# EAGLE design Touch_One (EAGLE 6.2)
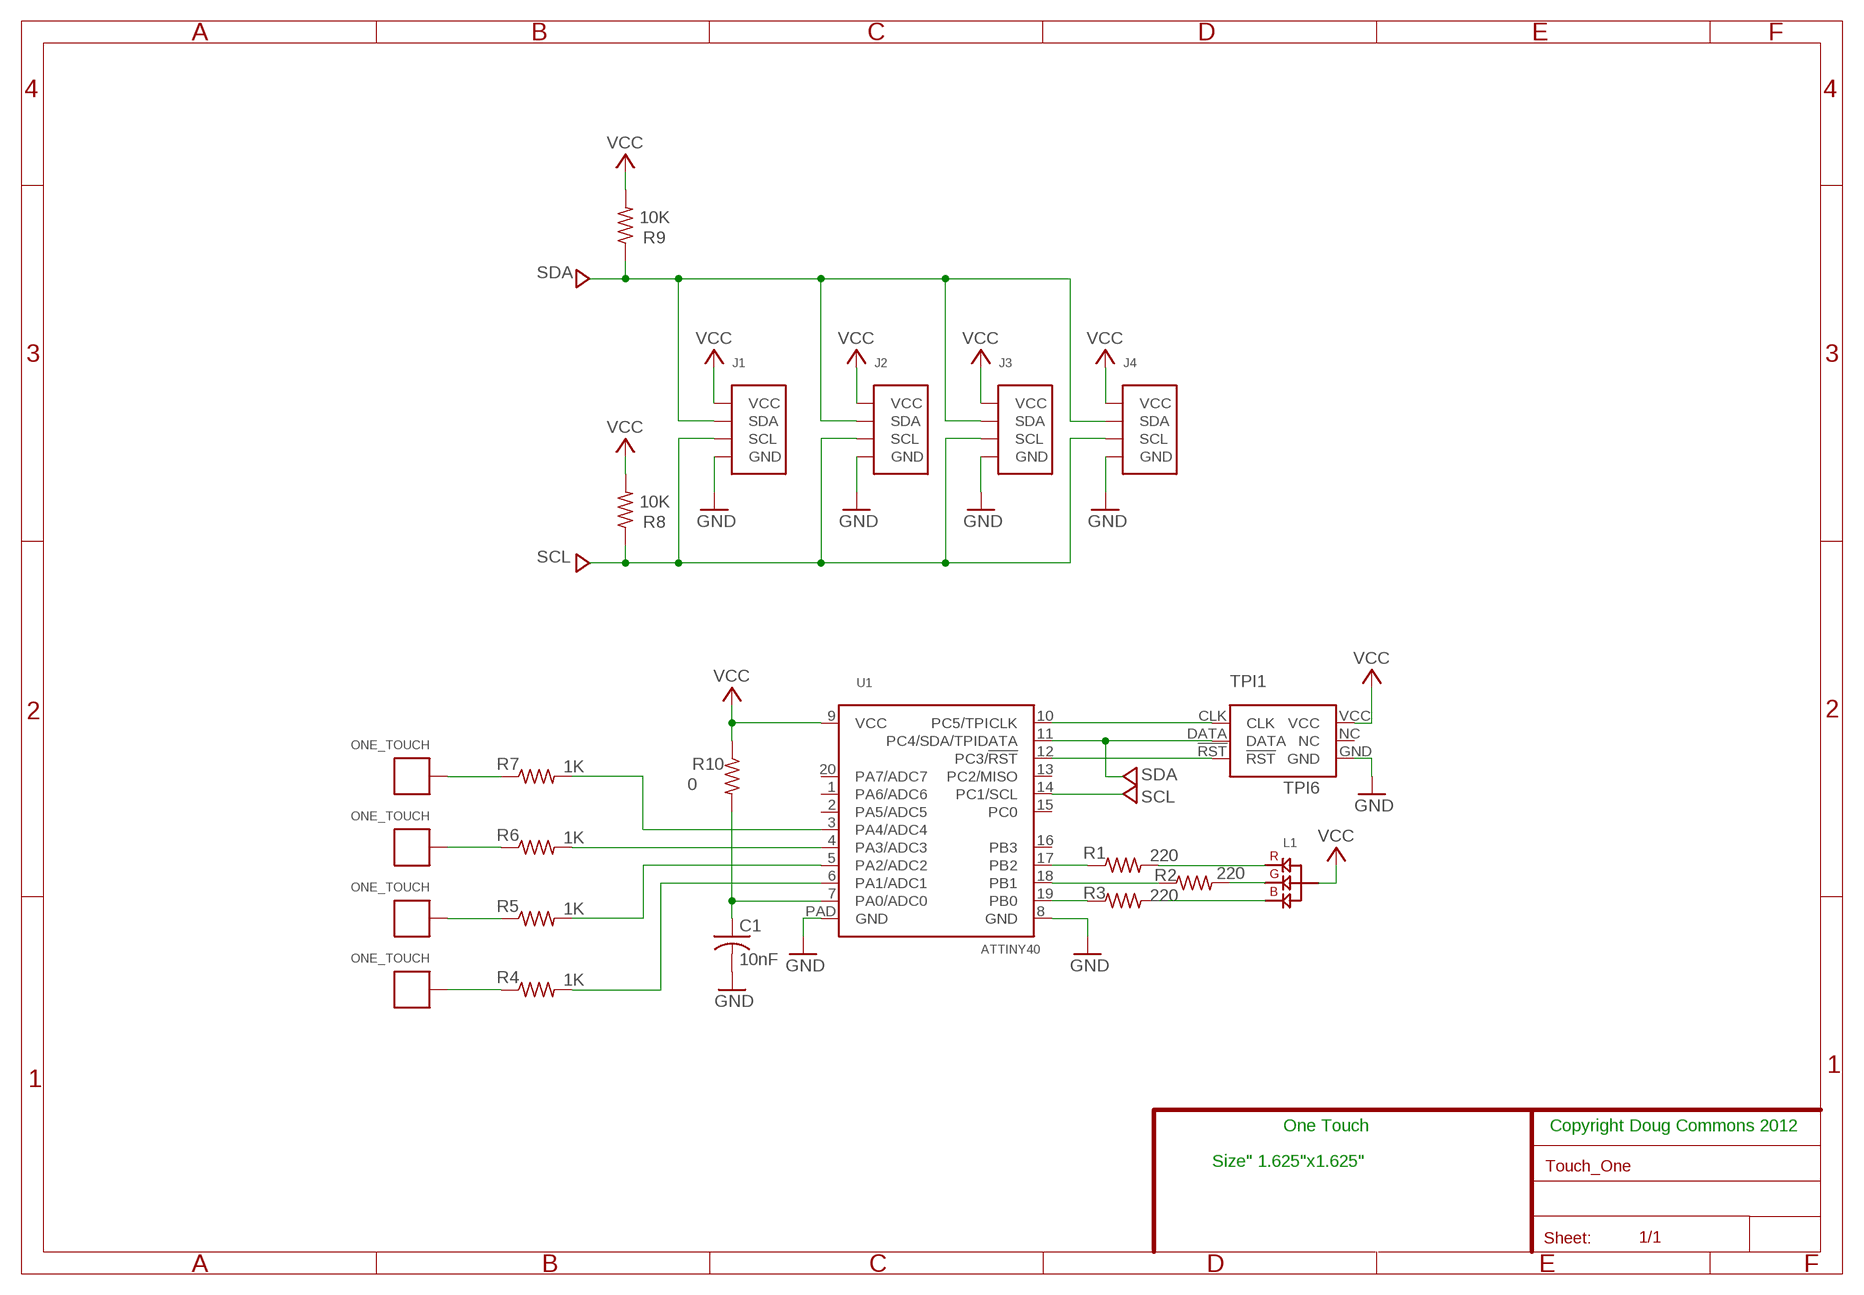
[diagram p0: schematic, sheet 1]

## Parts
C1  10nF  C-USC0805  [C0805]
J1  I44  [I44]
J2  I44R  [I44R]
J3  I44R  [I44R]
J4  I44  [I44]
L1  RGB_ANODE  [3.2X2.7]
R1  220  R-US_R0805  [R0805]
R2  220  R-US_R0805  [R0805]
R3  220  R-US_R0805  [R0805]
R4  1K  R-US_R0805  [R0805]
R5  1K  R-US_R0805  [R0805]
R6  1K  R-US_R0805  [R0805]
R7  1K  R-US_R0805  [R0805]
R8  10K  R-US_R0805  [R0805]
R9  10K  R-US_R0805  [R0805]
R10  0  R-US_R0805  [R0805]
SW1  ONE_TOUCH  [ONE_TOUCH]
SW2  ONE_TOUCH  [ONE_TOUCH]
SW3  ONE_TOUCH  [ONE_TOUCH]
SW4  ONE_TOUCH  [ONE_TOUCH]
TPI1  TPI6  [TPI6]
U1  ATTINY40  [VQFN20]

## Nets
GND: C1.2 J1.GND J2.GND J3.GND J4.GND TPI1.GND U1.8(GND) U1.PAD(GND)
N$1: TPI1.!RST U1.12(PC3/!RST)
N$2: R3.1 U1.19(PB0)
N$3: R2.1 U1.18(PB1)
N$4: L1.G R2.2
N$5: L1.R R1.2
N$6: L1.B R3.2
N$7: R7.1 SW4.P$1
N$8: R6.1 SW3.P$1
N$9: R5.1 SW2.P$1
N$10: R4.1 SW1.P$1
N$11: R4.2 U1.6(PA1/ADC1)
N$12: R5.2 U1.5(PA2/ADC2)
N$13: R6.2 U1.4(PA3/ADC3)
N$14: R7.2 U1.3(PA4/ADC4)
N$15: C1.1 R10.2 U1.7(PA0/ADC0)
N$17: TPI1.CLK U1.10(PC5/TPICLK)
N$18: R1.1 U1.17(PB2)
SCL: J1.SCL J2.SCL J3.SCL J4.SCL R8.1 U1.14(PC1/SCL)
SDA: J1.SDA J2.SDA J3.SDA J4.SDA R9.1 TPI1.DATA U1.11(PC4/SDA/TPIDATA)
VCC: J1.+5V(VCC) J2.+5V(VCC) J3.+5V(VCC) J4.+5V(VCC) L1.A R8.2 R9.2 R10.1 TPI1.VCC U1.9(VCC)
Unconnected: TPI1.NC U1.1(PA6/ADC6) U1.2(PA5/ADC5) U1.13(PC2/MISO) U1.15(PC0) U1.16(PB3) U1.20(PA7/ADC7)

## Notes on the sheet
- One Touch | Copyright Doug Commons 2012
- Size" 1.625"x1.625"

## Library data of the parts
C1 = 1_Dougs_custom:C-US: CAPACITOR, American symbol
J1 J4 = 1_Dougs_custom:I44
J2 J3 = 1_Dougs_custom:I44R
L1 = 1_Dougs_custom:RGB_ANODE
R1-R10 = 1_Dougs_custom:R-US_: RESISTOR, American symbol
SW1-SW4 = 1_Dougs_custom:ONE_TOUCH
TPI1 = 1_Dougs_custom:TPI6
U1 = 1_Dougs_custom:ATTINY40

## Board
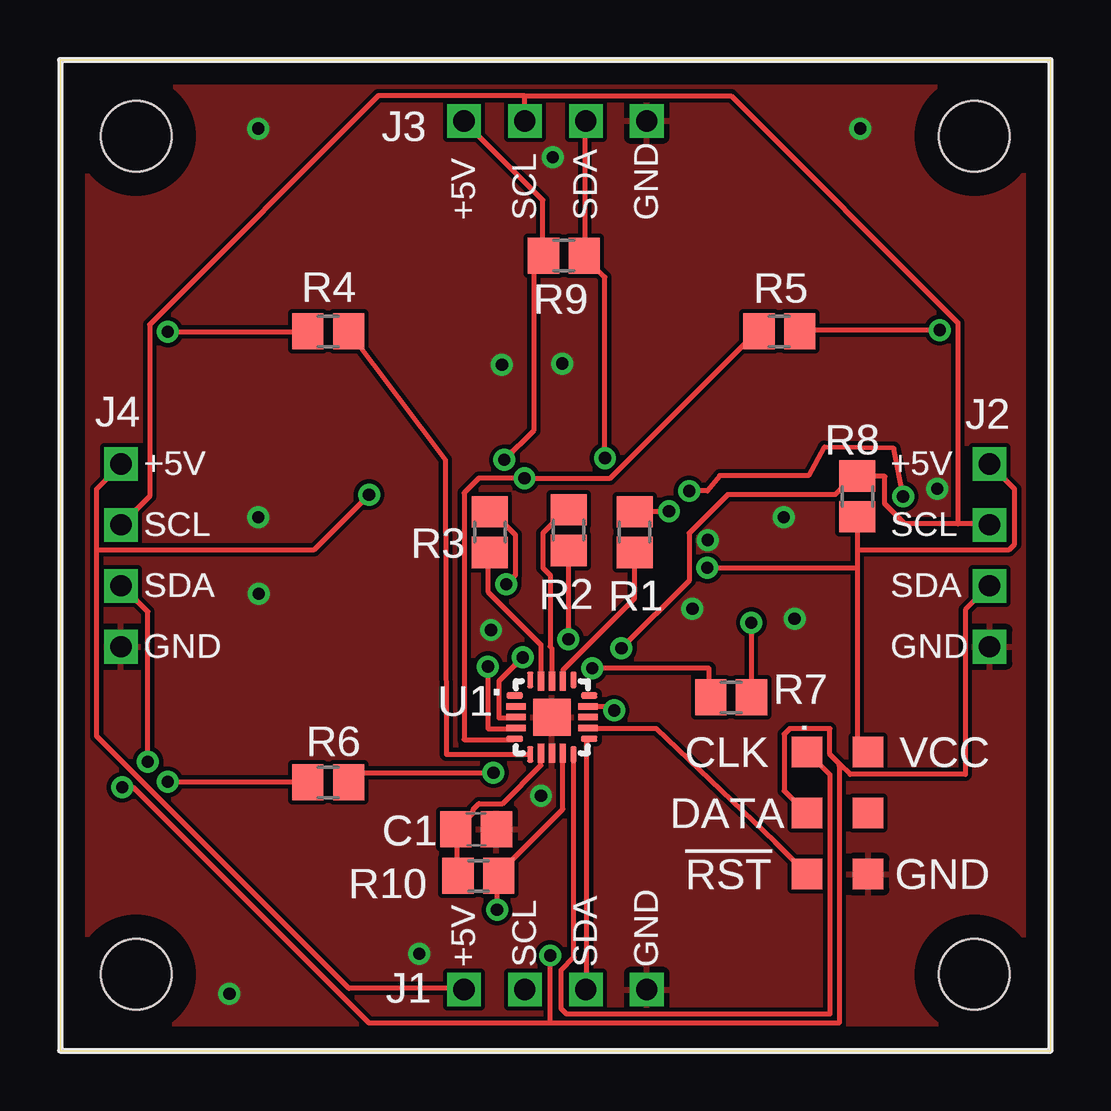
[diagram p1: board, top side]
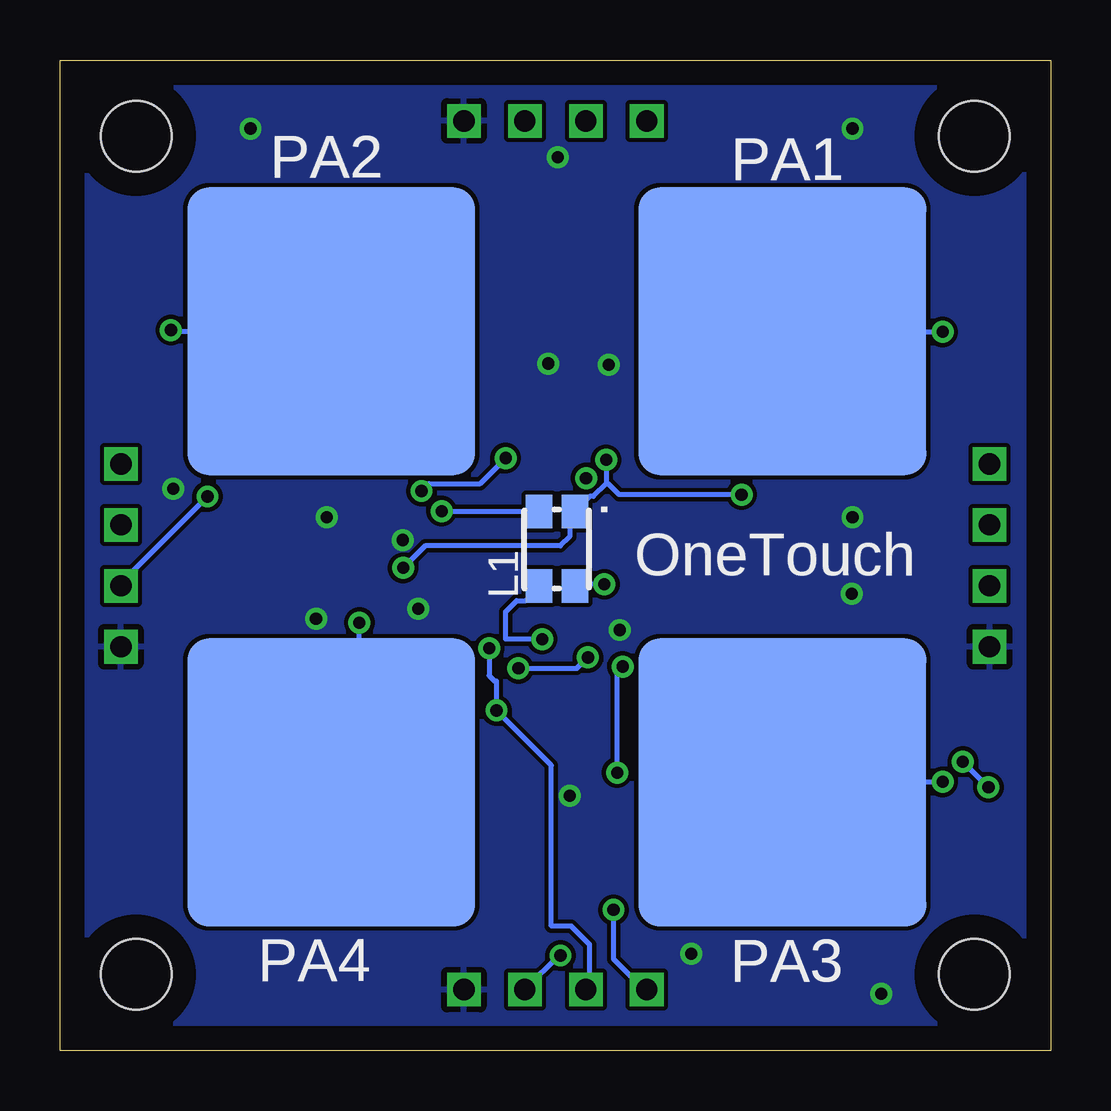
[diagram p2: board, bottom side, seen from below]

Size 41.27 x 41.27 mm. Coordinates in mm from the lower left corner, seen from the top.
Outline: 0,0 41.27,0 41.27,41.27 0,41.27 0,0
Copper layers (1*16): Top 0.035mm / dielectric 1.5mm / Bottom 0.035mm
Design rules: minimum track width 8mil, minimum drill 20mil, track to track 7mil, track to pad 7mil, pad to pad 7mil, via to via 7mil, smd to smd 0mil, copper to edge 40mil, drill to drill 10mil, minimum pad ring 10mil, minimum via ring 8mil, stop-mask expansion 0mil, vias tented up to drill 0mil, thermal gap 10mil
Holes 2.95 mm at 3.17,3.17 38.1,3.17 38.1,38.1 3.17,38.1

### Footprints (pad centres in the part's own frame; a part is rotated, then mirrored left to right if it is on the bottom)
C0805 = smd 1.3 x 1.5: 1 -0.85,0; 2 0.85,0
I44 = drill 0.889 square: +5V 0,3.81; GND 0,-3.81; SCL 0,1.27; SDA 0,-1.27
I44R = drill 0.889 square: +5V 0,3.81; GND 0,-3.81; SCL 0,1.27; SDA 0,-1.27
3.2X2.7 = smd 1.4 x 1.1: A 1.55,-0.75; B -1.55,-0.75; G -1.55,0.75; R 1.55,0.75
R0805 = smd 1.3 x 1.5: 1 -0.85,0; 2 0.85,0
ONE_TOUCH = smd 12 x 12: P$1 0,0
TPI6 = smd 1.27 x 1.27: !RST 2.54,-1.27; CLK -2.54,-1.27; DATA 0,-1.27; GND 2.54,1.27; NC 0,1.27; VCC -2.54,1.27
VQFN20 = smd 0.7 x 0.27: 1 -1.55,0.9; 5 -1.55,-0.9; 11 1.55,-0.9; 15 1.55,0.9 | smd 0.8 x 0.27: 2 -1.5,0.45; 3 -1.5,0; 4 -1.5,-0.45; 12 1.5,-0.45; 13 1.5,0; 14 1.5,0.45 | smd 0.27 x 0.7: 6 -0.9,-1.55; 10 0.9,-1.55; 16 0.9,1.55; 20 -0.9,1.55 | smd 0.27 x 0.8: 7 -0.45,-1.5; 8 0,-1.5; 9 0.45,-1.5; 17 0.45,1.5; 18 0,1.5; 19 -0.45,1.5 | smd 1.55 x 1.55: PAD 0,0

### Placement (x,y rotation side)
C1  17.34,9.22 0 top
J1  20.64,2.54 90 top
J2  38.73,20.64 0 top
J3  20.64,38.73 90 top
J4  2.54,20.64 0 top
L1  20.57,20.9 90 bottom
R1  23.94,21.6 90 top
R2  21.2,21.69 270 top
R3  17.91,21.6 90 top
R4  11.18,29.97 0 top
R5  29.97,29.97 180 top
R6  11.18,11.18 0 top
R7  27.97,14.72 180 top
R8  33.22,23.09 270 top
R9  20.99,33.12 180 top
R10  17.44,7.28 180 top
SW1  11.18,29.97 0 bottom
SW2  29.97,29.97 0 bottom
SW3  11.18,11.18 0 bottom
SW4  29.97,11.18 0 bottom
TPI1  32.4,9.89 270 top
U1  20.5,13.89 0 top

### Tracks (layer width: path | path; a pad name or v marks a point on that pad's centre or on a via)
GND  (via drill 0.51)
  Top 0.203: 20.42,13.18 U1.PAD 20.5,13.77
  other vias: 8.26,38.42 33.34,38.42 30.16,22.23 18.41,28.57 8.26,22.23 7.06,2.37 14.97,4.04 26.35,18.41 26.99,21.27 20.04,10.62 8.28,19.04 36.55,23.41 30.61,18 20.54,37.22 17.96,17.53 20.93,28.63
  pour Top: 0.1,41.29 41.34,41.39 41.34,0 0.05,0 0,41.34
  pour Bottom: -0.05,0.05 0,41.34 41.39,41.24 41.24,-0.05 0.1,0 0,-0.05
N$1
  Top 0.203: TPI1.!RST 29.79,8.69 24.84,13.41 22.02,13.41 U1.12
N$2
  Top 0.203: U1.19 20.04,15.47 20.04,16.92 17.83,19.13 17.83,20.65 17.91,20.73 R3.1
N$3
  Top 0.203: U1.18 20.5,16.76 20.42,16.84 20.42,19.81 20.12,20.12 20.12,21.57 21.03,22.48 21.18,22.48 R2.1
N$4  (via drill 0.51)
  Top 0.203: v21.18,17.14 21.18,20.8 R2.2
  Bottom 0.203: v21.18,17.14 22.71,17.14 22.71,18.29 22.25,18.75 21.87,18.75 21.34,19.28 L1.G
N$5  (via drill 0.51)
  Top 0.203: v25.38,22.48 24,22.48 R1.2
  Bottom 0.203: v25.38,22.48 21.34,22.48 L1.R
N$6  (via drill 0.51)
  Top 0.203: v18.59,19.43 18.97,19.81 18.97,21.49 18.06,22.4 17.91,22.4 R3.2
  Bottom 0.203: v18.59,19.43 19.74,19.43 L1.B
N$7  (via drill 0.51)
  Top 0.203: v28.8,17.83 28.8,14.78 R7.1
  Bottom 0.203: 30.1,11.2 30.02,11.2 SW4.P$1 30.02,11.28 28.8,11.28 v28.8,17.83
N$8  (via drill 0.51)
  Top 0.203: v4.5,11.2 10.29,11.2 R6.1
  Bottom 0.203: v4.5,11.2 11.12,11.2 SW3.P$1
N$9  (via drill 0.51)
  Top 0.203: v36.65,30.02 30.86,30.02 R5.1
  Bottom 0.203: v36.65,30.02 36.58,29.95 30.02,29.95 SW2.P$1
N$10  (via drill 0.51)
  Top 0.203: v4.5,29.95 10.29,29.95 R4.1
  Bottom 0.203: v4.5,29.95 11.12,29.95 SW1.P$1
N$11
  Top 0.203: U1.6 19.58,12.34 16.1,12.34 16.05,24.61 12.04,29.95 R4.2
N$12  (via drill 0.51)
  Top 0.203: U1.5 18.9,12.95 16.84,12.95 16.84,23.24 17.45,23.85 v19.36,23.85 22.94,23.85 29.03,29.95 R5.2 29.11,29.95
N$13  (via drill 0.51)
  Top 0.203: v17.83,16 17.83,13.41 18.97,13.41 U1.4 | v18.06,11.58 12.04,11.58 12.04,11.2 R6.2
  Bottom 0.203: v17.83,16 18.06,15.77 v18.06,11.58
N$14  (via drill 0.51)
  Top 0.203: v19.28,16.38 18.29,15.39 18.29,13.87 18.97,13.87 U1.3 | v22.17,15.93 27.05,15.93 27.05,14.78 R7.2
  Bottom 0.203: v19.28,16.38 19.74,15.93 v22.17,15.93
N$15
  Top 0.203: U1.7 20.04,12.34 20.04,11.89 18.44,10.29 17.45,10.29 17.22,10.06 17.22,9.91 16.54,9.22 C1.1 16.54,9.14 16.54,7.32 R10.2
N$17
  Top 0.203: U1.10 21.41,12.27 21.41,3.89 20.88,3.35 20.88,1.75 21.11,1.52 32.08,1.52 32.08,11.51 31.17,12.42 TPI1.CLK
N$18
  Top 0.203: U1.17 20.95,15.47 20.95,15.85 23.93,18.82 23.93,20.73 R1.1
SCL  (via drill 0.51)
  Top 0.203: v23.09,14.17 23.09,14.33 22.02,14.33 U1.14 | 37.41,21.95 38.71,21.95 J2.SCL | 37.41,21.95 35.2,21.95 34.37,22.78 34.37,23.93 33.22,23.93 R8.1 33.15,24 32.31,23.16 27.81,23.16 26.21,21.57 26.21,19.58 v23.39,16.76 | 19.36,39.78 13.26,39.78 3.73,30.25 3.73,23.09 2.59,21.95 J4.SCL | 19.36,39.78 19.36,38.79 J3.SCL | 37.41,21.95 37.41,30.33 27.96,39.78 19.36,39.78
  Bottom 0.203: J1.SCL 19.36,2.59 19.2,2.59 19.2,4.42 19.96,5.18 20.8,5.18 20.8,11.89 v23.09,14.17 23.09,15.39 23.16,15.39 23.39,15.62 v23.39,16.76
SDA  (via drill 0.51)
  Top 0.203: J3.SDA 21.87,38.71 21.87,33.15 R9.1 21.87,33.07 22.71,32.23 v22.71,24.69 | U1.11 22.02,12.95 21.95,12.88 21.95,2.59 J1.SDA | 32.5,11.93 32.92,11.51 37.72,11.51 37.72,18.36 38.71,19.36 J2.SDA | 32.5,11.93 32.08,12.34 32.08,13.41 30.4,13.41 30.18,13.18 30.18,10.82 31.09,9.91 TPI1.DATA | v3.66,12.04 3.66,18.29 2.59,19.36 J4.SDA | v2.59,10.97 3.05,10.97 12.88,1.14 20.42,1.14 | 20.42,1.14 32.46,1.14 32.46,11.89 32.5,11.93 | v35.13,23.09 34.75,25.09 31.85,25.15 31.19,23.95 27.48,23.95 26.98,23.32 v26.21,23.32 | 20.42,1.14 v20.42,3.96
  Bottom 0.203: v2.59,10.97 v3.66,12.04 | v35.13,23.09 38.79,19.43 J2.SDA | v20.42,3.96 20.5,3.96 21.87,2.59 J1.SDA | v22.71,24.69 23.77,23.62 25.91,23.62 v26.21,23.32
VCC  (via drill 0.51)
  Top 0.203: v18.52,24.61 19.74,25.83 19.74,32.69 20.12,33.07 R9.2 20.12,33.15 20.12,35.43 16.84,38.71 J3.+5V | 1.52,20.88 1.52,13.11 12.04,2.59 16.76,2.59 J1.+5V | 1.52,20.88 1.52,23.39 2.52,24.38 J4.+5V | v12.88,23.16 10.59,20.88 1.52,20.88 | U1.9 20.95,12.34 20.95,10.06 18.29,7.39 18.29,7.32 R10.1 18.21,7.24 v18.21,5.87 | TPI1.VCC 33.22,12.88 33.22,20.12 | R8.2 33.22,20.88 | 33.22,20.88 33.22,20.12 | 33.22,20.88 39.55,20.88 39.78,21.11 39.78,23.39 38.79,24.38 J2.+5V | v26.98,20.12 33.22,20.12
  Bottom 0.203: 18.52,23.62 19.05,23.09 19.2,23.09 19.81,22.48 L1.A 19.89,22.4 20.04,22.4 20.04,21.41 20.42,21.03 26.06,21.03 v26.98,20.12 | v18.52,24.61 18.52,23.62 | v12.88,23.16 17.98,23.16 18.44,23.62 18.52,23.62 | v18.21,5.87 18.21,3.81 16.99,2.59 16.84,2.59 J1.+5V

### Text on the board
bPlace: PA1 | PA2 | OneTouch | PA3 | PA4
_tplace: J3 | +5V | SCL | SDA | GND | R9 | R5 | R4 | J4 | J2 | R8 | +5V | +5V | R3 | SCL | SCL | R1 | SDA | SDA | R2 | GND | R7 | GND | . | U1 | . | VCC | R6 | CLK | C1 | DATA | R10 | GND | !RST | +5V | SCL | SDA | GND | J1
_bplace: PA1 | PA2 | . | OneTouch | L1 | PA3 | PA4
